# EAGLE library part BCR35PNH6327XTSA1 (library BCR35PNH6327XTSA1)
Bipolar Transistors - Pre-Biased AF DIGITAL TRANSISTOR Source: Datasheet
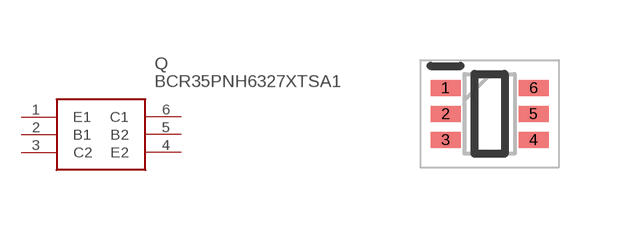
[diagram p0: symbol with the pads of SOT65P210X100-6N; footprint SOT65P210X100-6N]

Designator prefix Q

## BCR35PNH6327XTSA1 (Description: Bipolar Transistors - Pre-Biased AF DIGITAL TRANSISTOR; Height: 1mm; Manufacturer_Name: Infineon; Manufacturer_Part_Number: BCR35PNH6327XTSA1; Mouser_Part_Number: 726-BCR35PNH6327XTSA; Mouser_Price-Stock: https://www.mouser.com/Search/Refine.aspx?Keyword=726-BCR35PNH6327XTSA)  [SOT65P210X100-6N]
1  E1
2  B1
3  C2
4  E2
5  B2
6  C1

## Footprint SOT65P210X100-6N (pad centres in mm)
SOT363_
smd 0.75 x 0.4: 1 -1.1,0.65; 2 -1.1,0; 3 -1.1,-0.65; 4 1.1,-0.65; 5 1.1,0; 6 1.1,0.65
